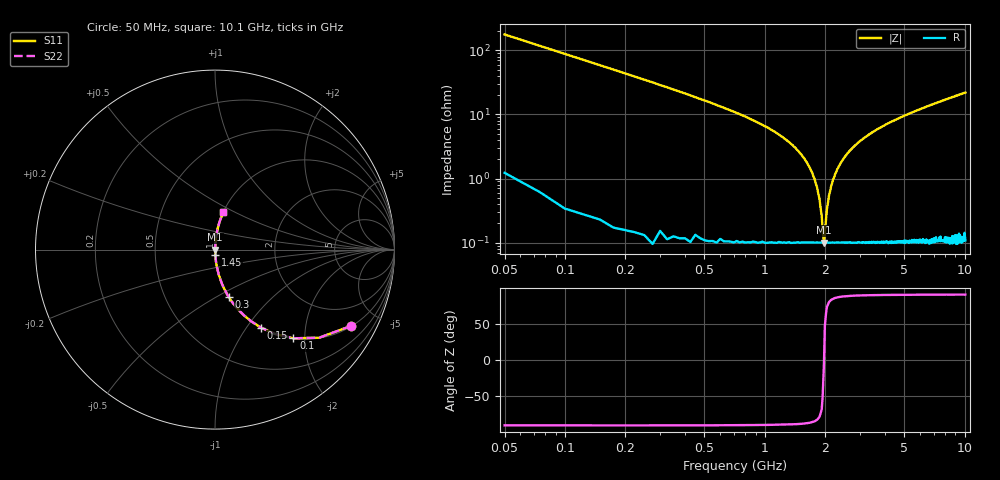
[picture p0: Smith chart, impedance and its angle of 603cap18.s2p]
! AVX Thin Film Operation		Date: November 2004
! Description: Accu-P® Series, Thin Film, SMD, RF Capacitor
! Part Number: 06033J180FBT
! 50 MHz  -  10.05 GHz
! Serial Measurements
# hz S db R 50
!	S11		S21		S12		S22
!	dB	Phase	dB	Phase	dB	Phase	dB	Phase
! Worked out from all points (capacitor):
!   400 points, 50 MHz to 10.1 GHz, reference 50 ohm
!   read as one part in series: C = 18 pF near 100 MHz
!   lowest |Z| = 100 mohm at 1.98 GHz (marker M1)
!   series resonance near 1.982 GHz, so ESL is about 360 pH
!   S11 on the Smith chart (normalised r, x): 50 MHz: 1.02, -3.54; 100 MHz: 1.01, -1.76; 150 MHz: 1.00, -1.17; 300 MHz: 1.00, -0.57; 1.45 GHz: 1.00, -0.06; 10.1 GHz: 1.00, +0.44
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5e7  -1.23 -29.4  -6.18 60.2  -6.18 60.2  -1.23 -29.4
1e8  -3.61 -48.5  -2.52 41.3  -2.52 41.3  -3.61 -48.5
1.5e8  -5.94 -59.5  -1.30 30.3  -1.30 30.3  -5.94 -59.5
3e8  -11.20 -73.7  -0.36 16.0  -0.36 16.0  -11.20 -73.7
6.75e8  -18.80 -82.9  -0.07 6.6  -0.07 6.6  -18.80 -82.9
1.45e9  -31.00 -86.3  -0.01 1.6  -0.01 1.6  -31.00 -86.3
1.73e9  -38.20 -84.6  -0.01 0.7  -0.01 0.7  -38.20 -84.6
1.83e9  -42.80 -81.6  -0.01 0.4  -0.01 0.4  -42.80 -81.6
1.88e9  -46.30 -77.8  -0.01 0.3  -0.01 0.3  -46.30 -77.8
1.93e9  -51.70 -67.2  -0.01 0.1  -0.01 0.1  -51.70 -67.2
1.95e9  -56.00 -50.9  -0.01 0.1  -0.01 0.1  -56.00 -50.9
1.98e9  -60.00 -5.5  -0.01 0.0  -0.01 0.0  -60.00 -5.5
2.05e9  -49.40 72.7  -0.01 -0.2  -0.01 -0.2  -49.40 72.7
2.1e9  -45.20 79.2  -0.01 -0.3  -0.01 -0.3  -45.20 79.2
2.2e9  -40.30 83.5  -0.01 -0.5  -0.01 -0.5  -40.30 83.5
2.3e9  -37.30 85.0  -0.01 -0.8  -0.01 -0.8  -37.30 85.0
2.65e9  -31.50 86.3  -0.01 -1.5  -0.01 -1.5  -31.50 86.3
3.4e9  -25.90 86.0  -0.02 -2.9  -0.02 -2.9  -25.90 86.0
5.08e9  -20.30 83.8  -0.05 -5.6  -0.05 -5.6  -20.30 83.8
6.75e9  -17.20 81.6  -0.09 -7.9  -0.09 -7.9  -17.20 81.6
8.43e9  -15.00 79.5  -0.15 -10.2  -0.15 -10.2  -15.00 79.5
1.01e10  -13.40 77.4  -0.21 -12.3  -0.21 -12.3  -13.40 77.4
